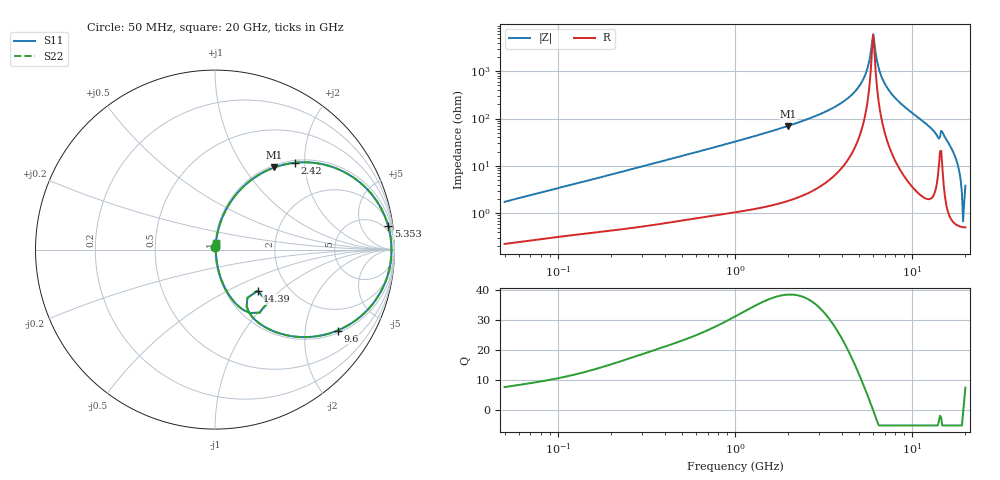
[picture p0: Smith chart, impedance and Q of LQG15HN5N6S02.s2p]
!Murata Part Number: LQG15HN5N6S02
!These Parameters are Measured in Series Mode Connection
!  o--[Z]--o
!Port1  Port2
!  o-------o
!Freq. Start=50[MHz] Stop=20[GHz], 401[Steps]
# Hz S RI R 50
!Freq.(Hz) S11(Real) S11(Imag) S21(Real) S21(Imag) S12(Real) S12(Imag) S22(Real) S22(Imag)
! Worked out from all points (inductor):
!   401 points, 50 MHz to 20 GHz, reference 50 ohm
!   read as one part in series: L = 5.46 nH near 51.52 MHz
!   highest Q = 38.3 at 1.992 GHz (marker M1), where L = 5.57 nH
!   self-resonance near 5.944 GHz
!   S11 on the Smith chart (normalised r, x): 50 MHz: 1.00, +0.03; 2.42 GHz: 1.05, +1.79; 5.353 GHz: 3, +14; 9.6 GHz: 1.09, -2.97; 14.39 GHz: 1.40, -0.73; 20 GHz: 1.01, +0.08
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5e7  0.00255 0.0173  0.9975 -0.0173  0.9975 -0.0173  0.00255 0.0173
1.364002e8  0.00566 0.0449  0.9943 -0.0449  0.9943 -0.0449  0.00566 0.0449
3.721004e8  0.02 0.1176  0.98 -0.1176  0.98 -0.1176  0.02 0.1176
1e9  0.1032 0.2885  0.8968 -0.2885  0.8968 -0.2885  0.1032 0.2885
1.99176e9  0.331 0.4577  0.669 -0.4577  0.669 -0.4577  0.331 0.4577
2.419936e9  0.4455 0.4839  0.5545 -0.4839  0.5545 -0.4839  0.4455 0.4839
2.728004e9  0.5273 0.4855  0.4727 -0.4855  0.4727 -0.4855  0.5273 0.4855
4.212059e9  0.8472 0.3373  0.1528 -0.3373  0.1528 -0.3373  0.8472 0.3373
4.81993e9  0.925 0.2308  0.075 -0.2308  0.075 -0.2308  0.925 0.2308
5.352748e9  0.9657 0.1295  0.0343 -0.1295  0.0343 -0.1295  0.9657 0.1295
6.034176e9  0.9835 -0.000585  0.0165 0.000585  0.0165 0.000585  0.9835 -0.000585
6.701223e9  0.9686 -0.1203  0.0314 0.1203  0.0314 0.1203  0.9686 -0.1203
7.442007e9  0.9222 -0.2373  0.0778 0.2373  0.0778 0.2373  0.9222 -0.2373
9.600142e9  0.6826 -0.4509  0.3174 0.4509  0.3174 0.4509  0.6826 -0.4509
1.201863e10  0.3748 -0.471  0.6252 0.471  0.6252 0.471  0.3748 -0.471
1.375312e10  0.1901 -0.3512  0.8099 0.3512  0.8099 0.3512  0.1901 -0.3512
1.438523e10  0.2374 -0.23  0.7626 0.23  0.7626 0.23  0.2374 -0.23
1.527346e10  0.1608 -0.338  0.8392 0.338  0.8392 0.338  0.1608 -0.338
1.721783e10  0.0379 -0.1744  0.9621 0.1744  0.9621 0.1744  0.0379 -0.1744
1.828096e10  0.0135 -0.0894  0.9865 0.0894  0.9865 0.0894  0.0135 -0.0894
1.912117e10  0.00576 -0.0256  0.9942 0.0256  0.9942 0.0256  0.00576 -0.0256
2e10  0.00644 0.0375  0.9936 -0.0375  0.9936 -0.0375  0.00644 0.0375
